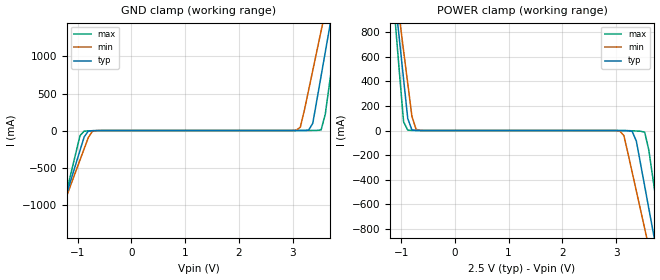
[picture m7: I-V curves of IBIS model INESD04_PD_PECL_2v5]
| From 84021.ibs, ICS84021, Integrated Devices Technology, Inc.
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[Model] INESD04_PD_PECL_2v5
Model_type   Input
Polarity   Non-Inverting
Vinl = 0.7V
Vinh = 1.7V
|   typ   min   max
C_comp   2pF   1.5pF   2.5pF
|   typ   min   max
[Voltage range]  2.5V   2.375V   2.625V
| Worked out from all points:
|   GND clamp passes 1 mA (typ) near -0.66 V on its own axis
|   POWER clamp passes 1 mA (typ) near -0.73 V on its own axis
[GND_clamp]
|Voltage I(typ)   I(min)   I(max)
-2.5V     -3.923A    -3.439A    -4.738A
-1.418V   -1.364A    -1.309A    -1.47A
-953.6mV  -268mA     -397.3mA   -68.9mA
-876.3mV  -85.61mA   -245.7mA   -7.984mA
-644.3mV  -748.7uA   -1.017mA   -1.623mA
3.067V    77.99uA    3.842mA    46.62uA
3.144V    156.4uA    44.86mA    50.78uA
3.376V    97.83mA    812.2mA    527.9uA
3.531V    737mA      1.345A     8.592mA
3.686V    1.377A     1.877A     627.4mA
3.84V     2.018A     2.411A     1.446A
5V        6.827A     6.413A     7.596A
[POWER_clamp]
|Voltage   I(typ)   I(min)   I(max)
-2.5V     6.827A     5.981A     8.259A
-1.108V   1.057A     1.18A      879.9mA
-953.6mV  417.1mA    648.1mA    70.61mA
-876.3mV  97.83mA    382.1mA    3.299mA
-799mV    5.538mA    116.2mA    954.5uA
-644.3mV  156.4uA    914.3uA    117.2uA
3.067V    -251.8uA   -3.805mA   -50.04uA
3.299V    -6.93mA    -339.1mA   -2.143mA
3.531V    -450.5mA   -794.4mA   -13.06mA
3.686V    -815.6mA   -1.098A    -391.8mA
3.84V     -1.181A    -1.402A    -858.7mA
5V        -3.923A    -3.685A    -4.361A
